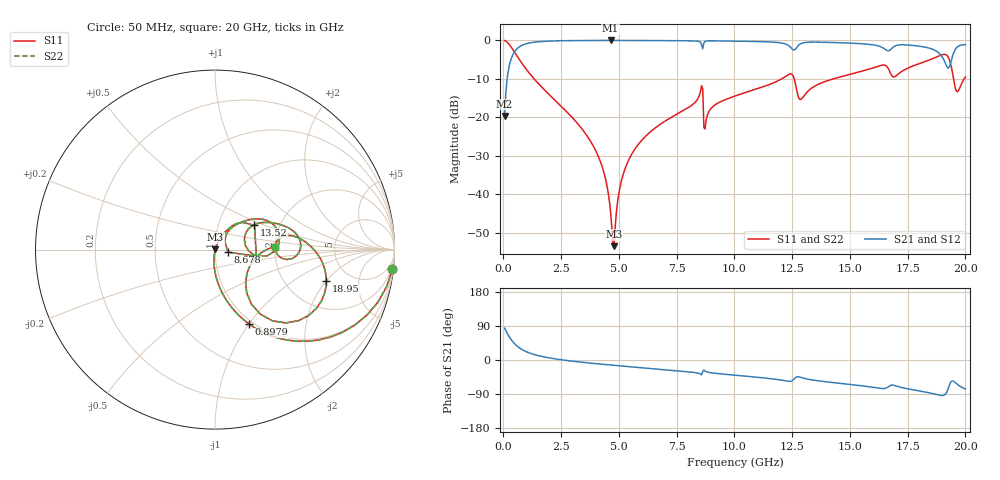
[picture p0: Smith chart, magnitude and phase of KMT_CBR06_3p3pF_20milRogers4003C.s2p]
! Data measured by Modelithics Inc. support@modelithics.com 813-866-6335
! KEMET CBR0603 3.3pF, Pad Width= 0.851mm, Pad Length= 0.64mm, Pad Gap= 0.62mm, 20mil Rogers 4003C substrate Data, January 2022
# hz S ma R 50
! 2 Port Network Data from SP1.SP block
! freq  magS11  angS11  magS21  angS21  magS12  angS12  magS22  angS22
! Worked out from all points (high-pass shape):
!   401 points, 50 MHz to 20 GHz, reference 50 ohm
!   highest |S21| = -0.02 dB at 4.638 GHz (marker M1); lowest = -19.7 dB at 50 MHz (marker M2)
!   |S21| within 3 dB of the highest: 475 MHz to 18.8 GHz (18.33 GHz wide, 190 % of centre); 19.51 GHz to end of sweep
!   lowest |S11| = -53.5 dB at 4.788 GHz (marker M3), VSWR 1.00, Z = 50.2 + j0.0609 ohm
!   |S11| at or under -10 dB: 1.327 GHz to 12.05 GHz (10.72 GHz wide, 160 % of centre); 12.59 GHz to 14.28 GHz (1.696 GHz wide, 12.6 % of centre); 19.49 GHz to 19.95 GHz (458 MHz wide, 2.32 % of centre)
!   |S22| runs from -53.5 to 0.0 dB; largest |S21 - S12| = 0
!   S11 on the Smith chart (normalised r, x): 50 MHz: 1, -19; 897.9 MHz: 0.96, -1.00; 8.678 GHz: 1.15, -0.03; 13.52 GHz: 1.48, +0.44; 18.95 GHz: 3.33, -2.02; 20 GHz: 2.00, +0.07
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5e7  0.9946 -6.1  0.104 83.9  0.104 83.9  0.9946 -6.1
3.4925e8  0.8058 -37.3  0.5913 52.7  0.5913 52.7  0.8058 -37.3
8.97875e8  0.4573 -65.3  0.8884 24.6  0.8884 24.6  0.4573 -65.3
3.391625e9  0.07109 -94.6  0.9958 -5.9  0.9958 -5.9  0.07109 -94.6
4.2395e9  0.02445 -97.0  0.9978 -11.0  0.9978 -11.0  0.02445 -97.0
4.6385e9  0.005885 -85.6  0.998 -13.3  0.998 -13.3  0.005885 -85.6
4.788125e9  0.002113 16.7  0.998 -14.1  0.998 -14.1  0.002113 16.7
5.33675e9  0.02445 68.5  0.9976 -17.0  0.9976 -17.0  0.02445 68.5
6.73325e9  0.07903 64.2  0.9944 -24.2  0.9944 -24.2  0.07903 64.2
8.52875e9  0.2158 44.8  0.9466 -37.2  0.9466 -37.2  0.2158 44.8
8.678375e9  0.07344 -11.0  0.9287 -26.4  0.9287 -26.4  0.07344 -11.0
1.0025e10  0.1891 48.9  0.9781 -40.1  0.9781 -40.1  0.1891 48.9
1.236912e10  0.3629 19.1  0.8448 -56.4  0.8448 -56.4  0.3629 19.1
1.286788e10  0.1704 14.4  0.9037 -45.7  0.9037 -45.7  0.1704 14.4
1.336662e10  0.2426 32.6  0.9497 -52.6  0.9497 -52.6  0.2426 32.6
1.351625e10  0.2582 32.4  0.9497 -54.0  0.9497 -54.0  0.2582 32.4
1.670825e10  0.4037 -7.9  0.7384 -68.7  0.7384 -68.7  0.4037 -7.9
1.78055e10  0.4742 7.6  0.8553 -79.4  0.8553 -79.4  0.4742 7.6
1.895262e10  0.645 -15.9  0.6361 -93.4  0.6361 -93.4  0.645 -15.9
1.930175e10  0.5673 -46.1  0.4487 -67.0  0.4487 -67.0  0.5673 -46.1
1.965088e10  0.2146 -25.1  0.8232 -64.0  0.8232 -64.0  0.2146 -25.1
2e10  0.3347 2.8  0.8811 -76.5  0.8811 -76.5  0.3347 2.8
